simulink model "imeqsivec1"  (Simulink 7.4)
settings: Solver=ode45  StartTime=0.0  StopTime=1  MaxStep=1e-3  RelTol=1e-3
InitFcn:
  | imdefsivec1
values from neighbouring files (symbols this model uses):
  Bm = 0.10    (= 0.1)    [IMabc2.m]    (also in imabcparam.m = 0.01; IMabcrun0.m = 0.01; IMabcrun1.m = 0.001; IMcur0.m = 1e-06)
  fr0 = [phidr phiqr]    [imdef0vec.m]    (also in imdef1vec.m; imdefrotflux.m = sqrt(phidr^2+phiqr^2); imdefSIvec1.m)
  fs0 = fs    [calc0.m]    (also in imdef0vec.m = [phids phiqs]; imdef1vec.m = [phids phiqs]; imdefrotflux.m = [fs0d fs0q]; imdefSIvec1.m = [phids phiqs])
  J = 0.02    [imabcparam.m]    (also in IMabcrun0.m; IMabcrun1.m; imdefSIvec1.m = 0.03)
  Lm = eval(get(hLm,'String'))    [im3d.m]    (also in IMabc2.m = 4.5; imabcparam.m = 0.0847; IMabcrun0.m = 0.0847; IMabcrun1.m = 0.0847)
  Lrl = eval(get(hLr,'String'))    [im3d.m]    (also in IMabc2.m = 0.1; imabcparam.m = 0.0025; IMabcrun0.m = 0.0025; IMabcrun1.m = 0.0025)
  Lsl = eval(get(hLs,'String'))    [im3d.m]    (also in IMabc2.m = 0.1; imabcparam.m = 0.0025; IMabcrun0.m = 0.0025; IMabcrun1.m = 0.0025)
  p = cos(beta-alpha)    [abcRwdg.m]    (also in alternator.m = 0:pi/20:2*pi; altwdgs.m = 0:pi/20:2*pi; brushlessdcB.m = 0:pi/100:2*pi; brushlessdcnew.m = 0:pi/100:2*pi)
  Rr = input('Rotor resistance)[default = 2] =')    [Actac.m]    (also in im1phase.m = 0.3; im3d.m = eval(get(hRr,'String')); IMabc2.m = 0.02; imabcparam.m = 0.408)
  Rs = eval(get(hRs,'String'))    [im3d.m]    (also in IMabc2.m = 0.01; imabcparam.m = 0.531; IMabcrun0.m = 0.531; IMabcrun1.m = 0.531)
  Tl0 = Is*conj(Is)*Req    [imdef0vec.m]    (also in imdef1vec.m; imdef2vec.m = Lm*(I(2)*I(3)-I(1)*I(4)); imdefrotflux.m; imdefSIvec1.m = Te0/To)
  To = 0.02    [fourier0.m]    (also in imdefSIvec1.m = 19.7882645911)
  Vo = Vll*sqrt(2/3)    [imdefSIvec1.m]
  vs = 1.0    (= 1)    [imdef0vec.m]    (also in imdef1vec.m; imdef2vec.m; imdefrotflux.m; imdefSIvec1.m)
  wk = ws    (= 1)    [imdef0vec.m]    (also in imdef1vec.m; imdef2vec.m; imdefrotflux.m; imdefSIvec1.m)
  wmec0 = n0*wo*2/p    (= 179.070781255)    [imdefSIvec1.m]
  wo = 2*pi*freq0    [calc0.m]    (also in IMabc2.m = 376.991118431; imabcparam.m = 376.991118431; IMabcrun0.m = 376.991118431; IMabcrun1.m = 376.991118431)

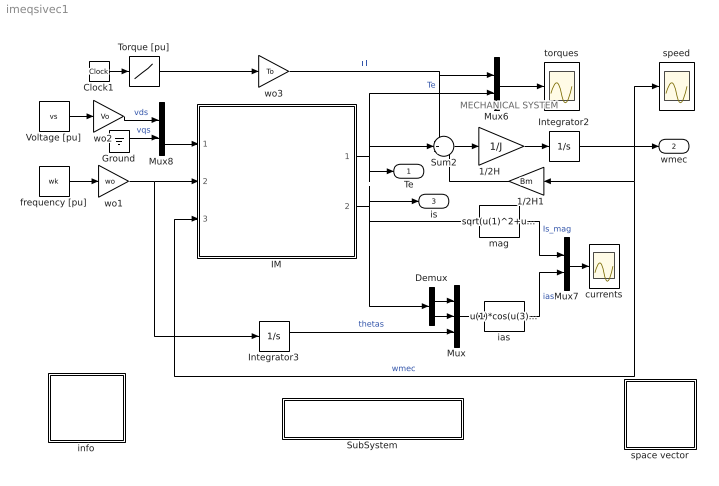
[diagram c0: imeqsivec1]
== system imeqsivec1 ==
  note: MECHANICAL SYSTEM
  1/2H : Gain  Gain=1/J  ParameterDataType=sfix(16)  ParameterScaling=2^0  OutDataType=sfix(16)  OutScaling=2^0
  1/2H1 : Gain  Gain=Bm  ParameterDataType=sfix(16)  ParameterScaling=2^0  OutDataType=sfix(16)  OutScaling=2^0
  Clock1 : Clock
  Demux : Demux  Outputs=2
  Ground : Ground
  IM : Subsystem
  Integrator2 : Integrator  InitialCondition=wmec0
  Integrator3 : Integrator
  Mux : Mux  Inputs=3
  Mux6 : Mux  Inputs=2
  Mux7 : Mux  Inputs=2
  Mux8 : Mux  Inputs=2
  SubSystem : Subsystem
  Sum2 : Sum  Inputs=-+-  OutDataType=sfix(16)  OutScaling=2^0
  Torque [pu] : Lookup  InputValues=[0 0.1 0.1 0.5 0.5 2]  Table="[Tl0 Tl0  0 0 0.5 0.5]"  OutDataType=sfix(16)  OutScaling=2^0
  Voltage [pu] : Constant  Value=vs  OutDataType=sfix(16)  OutScaling=2^0
  currents : Scope
  frequency [pu] : Constant  Value=wk  OutDataType=sfix(16)  OutScaling=2^0
  ias : Fcn  Expr=u(1)*cos(u(3))-u(2)*sin(u(3))
  info : Subsystem
  mag : Fcn  Expr=sqrt(u(1)^2+u(2)^2)
  space vector : Subsystem
  speed : Scope
  torques : Scope
  wo1 : Gain  Gain=wo  ParameterDataType=sfix(16)  ParameterScaling=2^0  OutDataType=sfix(16)  OutScaling=2^0
  wo2 : Gain  Gain=Vo  ParameterDataType=sfix(16)  ParameterScaling=2^0  OutDataType=sfix(16)  OutScaling=2^0
  wo3 : Gain  Gain=To  ParameterDataType=sfix(16)  ParameterScaling=2^0  OutDataType=sfix(16)  OutScaling=2^0
  Te : Outport
  wmec : Outport  Port=2
  is : Outport  Port=3
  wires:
  Demux/1 -> Mux/1
  Demux/2 -> Mux/2
  Mux/1 -> ias/1
  ias/1 -> Mux7/2  "ias"
  mag/1 -> Mux7/1  "Is_mag"
  Sum2/1 -> 1/2H/1
  1/2H/1 -> Integrator2/1
  Mux6/1 -> torques/1
  Clock1/1 -> Torque [pu]/1
  Torque [pu]/1 -> wo3/1
  wo3/1 -> Mux6/1, Sum2/1  "Tl"
  Mux8/1 -> IM/1(vs)
  Voltage [pu]/1 -> wo2/1
  wo2/1 -> Mux8/1  "vds"
  Ground/1 -> Mux8/2  "vqs"
  frequency [pu]/1 -> wo1/1
  wo1/1 -> Integrator3/1, IM/2(wk)
  Integrator3/1 -> Mux/3  "thetas"
  IM/1(Te) -> Sum2/2, Te/1, Mux6/2  "Te"
  IM/2(is) -> is/1, Demux/1, mag/1
  Integrator2/1 -> wmec/1, speed/1, 1/2H1/1, IM/3(wmec)  "wmec"
  Mux7/1 -> currents/1
  1/2H1/1 -> Sum2/3

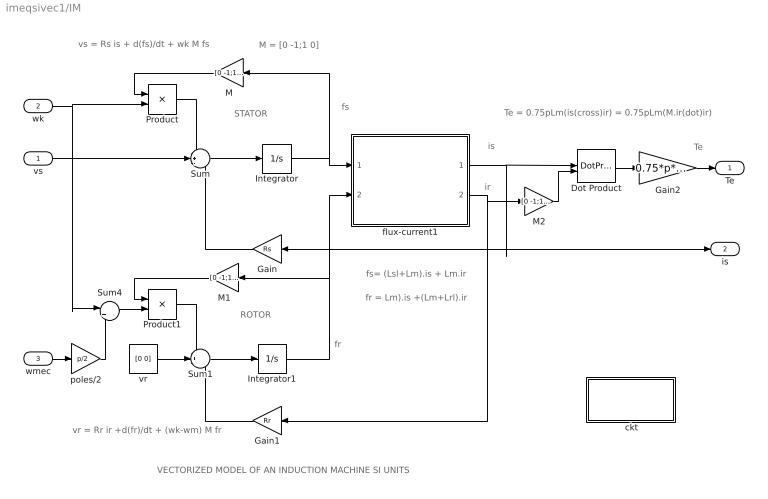
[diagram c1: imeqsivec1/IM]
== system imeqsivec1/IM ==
  note: ROTOR
  note: STATOR
  note: fs
  note: is
  note: Te
  note: VECTORIZED MODEL OF AN INDUCTION MACHINE SI UNITS
  note: vs = Rs is + d(fs)/dt + wk M fs
  note: vr = Rr ir +d(fr)/dt + (wk-wm) M fr
  note: fs= (Lsl+Lm).is + Lm.ir
  note: fr = Lm).is +(Lm+Lrl).ir
  note: Te = 0.75pLm(is(cross)ir) = 0.75pLm(M.ir(dot)ir)
  note: M = [0 -1;1 0]
  note: ir
  note: fr
  vs : Inport  OutDataType=sfix(16)  OutScaling=2^0
  wk : Inport  Port=2  OutDataType=sfix(16)  OutScaling=2^0
  wmec : Inport  Port=3  OutDataType=sfix(16)  OutScaling=2^0
  " ckt" : Subsystem
  Dot Product : DotProduct  OutDataType=fixdt(1, 16)  OutScaling=2^-10
  Gain : Gain  Gain=Rs  ParameterDataType=sfix(16)  ParameterScaling=2^0  OutDataType=sfix(16)  OutScaling=2^0
  Gain1 : Gain  Gain=Rr  ParameterDataType=sfix(16)  ParameterScaling=2^0  OutDataType=sfix(16)  OutScaling=2^0
  Gain2 : Gain  Gain=0.75*p*Lm  ParameterDataType=sfix(16)  ParameterScaling=2^0  OutDataType=sfix(16)  OutScaling=2^0
  Integrator : Integrator  InitialCondition=fs0
  Integrator1 : Integrator  InitialCondition=fr0
  M : Gain  Gain=[0 -1;1 0]  Multiplication=Matrix(K*u)  ParameterDataType=sfix(16)  ParameterScaling=2^0  OutDataType=sfix(16)  OutScaling=2^0
  M1 : Gain  Gain=[0 -1;1 0]  Multiplication=Matrix(K*u)  ParameterDataType=sfix(16)  ParameterScaling=2^0  OutDataType=sfix(16)  OutScaling=2^0
  M2 : Gain  Gain=[0 -1;1 0]  Multiplication=Matrix(K*u)  ParameterDataType=sfix(16)  ParameterScaling=2^0  OutDataType=sfix(16)  OutScaling=2^0
  Product : Product  OutDataType=sfix(16)  OutScaling=2^0
  Product1 : Product  OutDataType=sfix(16)  OutScaling=2^0
  Sum : Sum  Inputs=-+-  OutDataType=sfix(16)  OutScaling=2^0
  Sum1 : Sum  Inputs=-+-  OutDataType=sfix(16)  OutScaling=2^0
  Sum4 : Sum  Inputs=|+-  OutDataType=sfix(16)  OutScaling=2^0
  flux-current1 : Subsystem
  poles/2 : Gain  Gain=p/2  ParameterDataType=sfix(16)  ParameterScaling=2^0  OutDataType=sfix(16)  OutScaling=2^0
  vr : Constant  Value=[0 0]  OutDataType=sfix(16)  OutScaling=2^0
  Te : Outport
  is : Outport  Port=2
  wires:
  Gain/1 -> Sum/3
  vr/1 -> Sum1/2
  Gain1/1 -> Sum1/3
  Integrator/1 -> M/1, flux-current1/1(fs)
  Integrator1/1 -> flux-current1/2(fr), M1/1
  Product1/1 -> Sum1/1
  M1/1 -> Product1/1
  Product/1 -> Sum/1
  M/1 -> Product/1
  Sum4/1 -> Product1/2
  vs/1 -> Sum/2
  wk/1 -> Product/2, Sum4/1
  Sum1/1 -> Integrator1/1
  Sum/1 -> Integrator/1
  flux-current1/1(is) -> Gain/1, is/1, Dot Product/1
  Dot Product/1 -> Gain2/1
  Gain2/1 -> Te/1
  wmec/1 -> poles/2/1
  poles/2/1 -> Sum4/2
  M2/1 -> Dot Product/2
  flux-current1/2(ir) -> M2/1, Gain1/1

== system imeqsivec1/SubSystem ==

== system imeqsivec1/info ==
  note: The induction machine is modeled in vectorized form in conformity with the state vector formulation. This one-to-one correspondence can be seen by clicking both the INDUCTION MACHINE subsystem block and the MATHEMATICAL MODEL equation block. The synchronous reference frame is chosen here because the machine is operating under balanced three-phase sinusoidal excitation; the input voltage is thefore constant as indicated. The parameters describing the electromechanical system are expressed in SI units and may be modified by accessing an initialization m-file after clicking the bottom block. The system is initially assumed to be operated under load in a steady state defined by a specified speed. The initial conditions are established by performing a phasor calculation based on the standard steady-state equivalent circuit of the induction machine. In the present setup, the simulation portrays the dynamic response to a pulsed applied torque. The torque developed, the speed, and the stator current are observed on the scopes . The torque-speed dynamic characteristics can then be obtained after double clicking the X-Y PLOT block. Press start button.
  note: Running of a Line-Fed Induction Motor Synchronous frame SI units

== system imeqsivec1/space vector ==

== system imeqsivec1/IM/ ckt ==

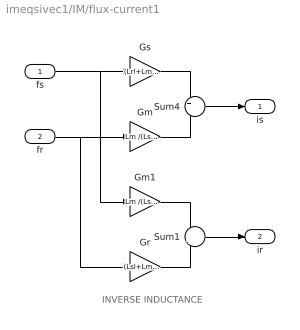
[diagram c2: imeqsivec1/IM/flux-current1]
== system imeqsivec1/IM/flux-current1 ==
  note: INVERSE INDUCTANCE
  fs : Inport  OutDataType=sfix(16)  OutScaling=2^0
  fr : Inport  Port=2  OutDataType=sfix(16)  OutScaling=2^0
  Gm : Gain  Gain=Lm /(Lsl*Lrl+Lsl*Lm+Lrl*Lm)  ParameterDataType=sfix(16)  ParameterScaling=2^0  OutDataType=sfix(16)  OutScaling=2^0
  Gm1 : Gain  Gain=Lm /(Lsl*Lrl+Lsl*Lm+Lrl*Lm)  ParameterDataType=sfix(16)  ParameterScaling=2^0  OutDataType=sfix(16)  OutScaling=2^0
  Gr : Gain  Gain=(Lsl+Lm )/(Lsl*Lrl+Lsl*Lm+Lrl*Lm)  ParameterDataType=sfix(16)  ParameterScaling=2^0  OutDataType=sfix(16)  OutScaling=2^0
  Gs : Gain  Gain=(Lrl+Lm) /(Lsl*Lrl+Lsl*Lm+Lrl*Lm)  ParameterDataType=sfix(16)  ParameterScaling=2^0  OutDataType=sfix(16)  OutScaling=2^0
  Sum1 : Sum  Inputs=-+  OutDataType=sfix(16)  OutScaling=2^0
  Sum4 : Sum  Inputs=+-  OutDataType=sfix(16)  OutScaling=2^0
  is : Outport
  ir : Outport  Port=2
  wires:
  fs/1 -> Gs/1, Gm1/1
  Gs/1 -> Sum4/1
  fr/1 -> Gm/1, Gr/1
  Gm/1 -> Sum4/2
  Sum4/1 -> is/1
  Gm1/1 -> Sum1/1
  Gr/1 -> Sum1/2
  Sum1/1 -> ir/1
